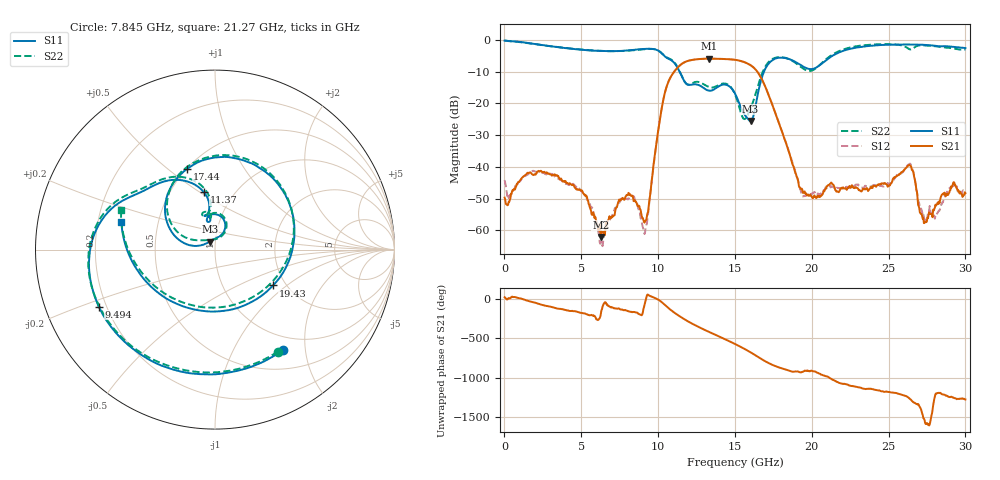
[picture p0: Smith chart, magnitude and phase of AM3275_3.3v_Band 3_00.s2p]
!Keysight Technologies,N5245B,MY58422270,A.16.20.02
!Date: Thursday, March 27, 2025 02:00:51
!Correction: S11(C  2-Port  )
!S21(C  2-Port  )
!S12(C  2-Port  )
!S22(C  2-Port  )
!S2P File: Measurements: S11, S21, S12, S22:
# Hz S  dB  R 50
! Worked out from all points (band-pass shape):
!   801 points, 10 MHz to 30 GHz, reference 50 ohm
!   highest |S21| = -5.95 dB at 13.32 GHz (marker M1); lowest = -62.0 dB at 6.27 GHz (marker M2)
!   |S21| within 3 dB of the highest: 11.24 GHz to 16.26 GHz (5.024 GHz wide, 36.5 % of centre)
!   lowest |S11| = -25.6 dB at 16.02 GHz (marker M3), VSWR 1.11, Z = 47.1 + j4.23 ohm
!   |S11| at or under -10 dB: 11.39 GHz to 16.9 GHz (5.505 GHz wide, 38.9 % of centre)
!   |S22| runs from -25.0 to -0.2 dB; largest |S21 - S12| = 0.0061
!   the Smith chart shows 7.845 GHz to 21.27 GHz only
!   S11 on the Smith chart (normalised r, x): 7.845 GHz: 0.78, -1.60; 9.494 GHz: 0.17, -0.23; 11.37 GHz: 0.73, +0.52; 17.44 GHz: 0.50, +0.59; 19.43 GHz: 1.72, -0.80; 21.27 GHz: 0.30, +0.13
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1e7  -0.28 -3.5  -49.69 22.4  -44.17 -50.0  -0.22 -4.6
1.247088e9  -0.83 -81.2  -42.93 -4.7  -43.25 -6.8  -0.87 -81.7
2.634125e9  -1.78 -159.6  -41.78 -84.1  -42.26 -81.2  -1.82 -160.7
5.033325e9  -3.15 86.3  -47.41 -176.4  -47.73 -179.1  -3.08 84.5
6.270412e9  -3.55 27.2  -62.04 166.5  -63.96 -56.1  -3.50 25.4
7.844888e9  -3.43 -55.9  -49.95 -139.1  -49.87 -137.2  -3.51 -58.3
9.119462e9  -2.88 -130.4  -57.55 -70.5  -61.12 139.8  -2.95 -132.9
9.494338e9  -2.83 -153.9  -48.43 36.6  -48.21 31.2  -2.88 -156.3
1.001916e10  -3.46 170.7  -28.19 -9.3  -28.14 -10.3  -3.42 168.5
1.136871e10  -9.77 100.9  -8.29 145.4  -8.28 145.3  -9.59 98.6
1.331806e10  -16.03 101.9  -5.95 -57.7  -5.95 -57.8  -14.87 97.3
1.5005e10  -16.94 66.1  -6.31 149.9  -6.31 149.8  -17.18 62.6
1.601716e10  -25.56 121.8  -8.01 44.3  -7.99 44.3  -21.54 141.7
1.744169e10  -6.44 108.8  -20.58 -114.9  -20.58 -115.0  -6.05 103.8
1.942852e10  -8.40 -31.7  -48.21 159.4  -49.34 163.4  -9.04 -38.1
2.002832e10  -9.22 -93.6  -49.56 168.7  -48.38 160.1  -9.65 -104.2
2.126541e10  -5.30 163.7  -44.94 68.5  -46.13 63.3  -4.93 157.4
2.298984e10  -2.41 91.7  -46.74 -37.1  -45.55 -35.8  -1.97 89.2
2.501416e10  -1.58 38.1  -46.02 -98.6  -45.28 -96.6  -1.40 34.6
2.64012e10  -1.50 4.3  -39.54 172.8  -38.99 172.4  -3.04 2.4
2.745085e10  -1.65 -23.5  -57.41 -144.4  -56.65 -144.5  -1.82 -23.7
3e10  -2.62 -112.1  -48.27 166.6  -47.30 -173.1  -3.10 -114.3
